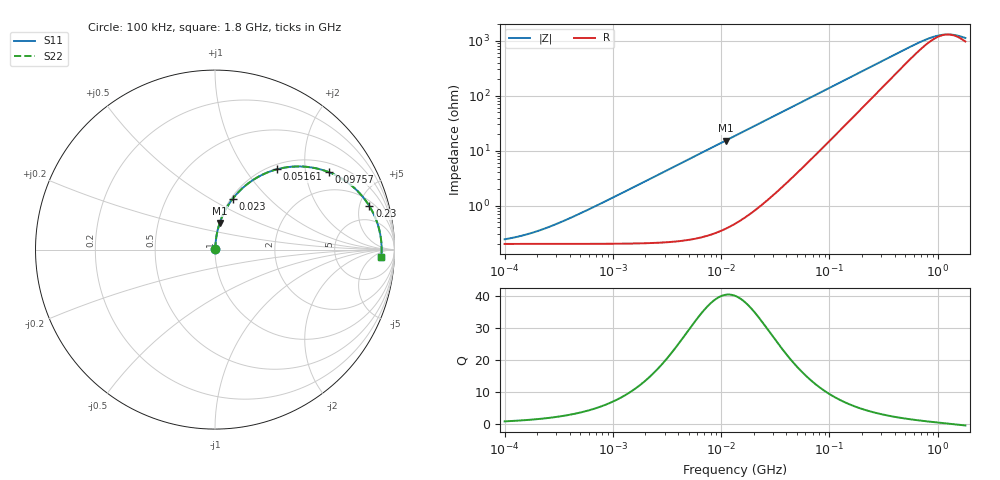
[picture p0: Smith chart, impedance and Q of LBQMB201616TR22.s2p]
! LBQMB201616TR22  S-PARAMETER MODEL  ( General Type )
! Model Generated by TAIYO YUDEN Corporation (http://www.ty-top.com)
! Version 1.0
! TAIYO YUDEN Control No. 191025NI43SB-FBB
! Copyright(c) 2019 TAIYO YUDEN CO.,LTD. All Rights Reserved.
! Product Description (link to TY-COMPAS)
! https://ds.yuden.co.jp/TYCOMPAS/or/detail?pn=LBQMB201616TR22J&u=M
! Products Name : Inductors
! Characteristics :
!  Inductance : 0.22 uH , SRF(min) : 450 MHz , DC Resistance(max) : 0.26 Ohm , Rated Current : 520 mA
!  Case Size : 2.0 x 1.6 / 0.079 x 0.063 [mm/inch] , Thickness : 1.6 / 0.063 [mm/inch]
!  (Conditions: Temperature = 25 degC , DC Bias Current/Voltage = 0A / 0V)
! External Node Assignments :
!  1  o---GGG---o  2
! GND o---------o GND
! Frequency Range : 0.1MHz  -  1800MHz  [ 402 STEP ]
# MHz S RI R 50
! Freq[MHz].  S11 Real  S11 Imag  S21 Real  S21 Imag  S12 Real  S12 Imag  S22 Real  S22 Imag
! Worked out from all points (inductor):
!   401 points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, 100 kHz to 1.8 GHz, reference 50 ohm
!   read as one part in series: L = 220 nH near 434.8 kHz
!   highest Q = 40.2 at 11.03 MHz (marker M1), where L = 220 nH
!   self-resonance near 1.236 GHz
!   S11 on the Smith chart (normalised r, x): 100 kHz: 1.00, +0.00; 23 MHz: 1.02, +0.64; 51.61 MHz: 1.08, +1.43; 97.57 MHz: 1.28, +2.69; 230 MHz: 2.57, +6.19; 1.8 GHz: 20, -11
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0.1  0.002 0.00138  0.998 -0.00138  0.998 -0.00138  0.002 0.00138
0.140908  0.002 0.00194  0.998 -0.00194  0.998 -0.00194  0.002 0.00194
0.208519  0.002 0.00287  0.998 -0.00287  0.998 -0.00287  0.002 0.00287
0.316224  0.00202 0.00435  0.998 -0.00435  0.998 -0.00435  0.00202 0.00435
0.516129  0.00205 0.00711  0.9979 -0.00711  0.9979 -0.00711  0.00205 0.00711
2.66389  0.00345 0.0366  0.9966 -0.0366  0.9966 -0.0366  0.00345 0.0366
5.833619  0.00891 0.0797  0.9911 -0.0797  0.9911 -0.0797  0.00891 0.0797
11.02886  0.0262 0.1479  0.9738 -0.1479  0.9738 -0.1479  0.0262 0.1479
13.41641  0.0374 0.1777  0.9626 -0.1777  0.9626 -0.1777  0.0374 0.1777
22.99727  0.0989 0.2836  0.9011 -0.2836  0.9011 -0.2836  0.0989 0.2836
34.03197  0.1909 0.3733  0.8091 -0.3733  0.8091 -0.3733  0.1909 0.3733
51.61028  0.3459 0.4476  0.6541 -0.4476  0.6541 -0.4476  0.3459 0.4476
69.24595  0.4799 0.4631  0.5201 -0.4631  0.5201 -0.4631  0.4799 0.4631
97.57284  0.6324 0.4321  0.3676 -0.4321  0.3676 -0.4321  0.6324 0.4321
147.9715  0.7735 0.3459  0.2265 -0.3459  0.2265 -0.3459  0.7735 0.3459
229.9669  0.8601 0.2424  0.1399 -0.2424  0.1399 -0.2424  0.8601 0.2424
357.3983  0.9018 0.1553  0.0982 -0.1553  0.0982 -0.1553  0.9018 0.1553
692.4421  0.9245 0.0615  0.0755 -0.0615  0.0755 -0.0615  0.9245 0.0615
975.7037  0.928 0.0241  0.072 -0.0241  0.072 -0.0241  0.928 0.0241
1130.179  0.9285 0.00903  0.0715 -0.00903  0.0715 -0.00903  0.9285 0.00903
1309.11  0.9285 -0.00582  0.0715 0.00582  0.0715 0.00582  0.9285 -0.00582
1800  0.927 -0.0388  0.073 0.0388  0.073 0.0388  0.927 -0.0388
